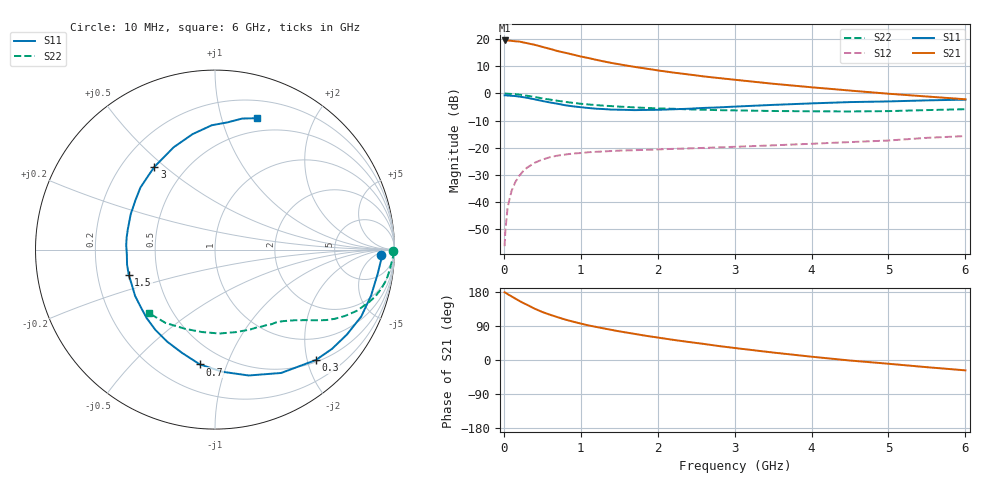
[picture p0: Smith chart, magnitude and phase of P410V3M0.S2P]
! SIEMENS Small Signal Semiconductors
! BFP182
! Si NPN RF Bipolar Junction Transistor in SOT143
! VCE = 10 V  IC = 3 mA
! Common Emitter S-Parameters:  March  1996
# GHz  S  MA  R  50
!  f  S11  S21  S12  S22
! GHz  MAG  ANG  MAG  ANG  MAG  ANG  MAG  ANG
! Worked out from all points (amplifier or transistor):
!   36 points, 10 MHz to 6 GHz, reference 50 ohm
!   highest |S21| = 19.6 dB at 10 MHz (marker M1)
!   |S21| within 3 dB of that: start of sweep to 585.2 MHz
!   unconditionally stable (mu >= 1): 2.001 GHz to 5.996 GHz
!   at 250 MHz: K = 0.16, MSG = 23.8 dB, |S12| = -28.8 dB
!   at 1.4 GHz: K = 0.76, MSG = 16.3 dB, |S12| = -21.3 dB
!   at 6 GHz: K = 1.00, MSG = 6.8 dB, |S12| = -15.8 dB
!   S11 on the Smith chart (normalised r, x): 10 MHz: 22, -8; 300 MHz: 0.54, -2.16; 700 MHz: 0.37, -0.81; 1.5 GHz: 0.34, -0.13; 3 GHz: 0.34, +0.46; 6 GHz: 0.36, +1.31
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0.01  0.9231 -1.7  9.558 178.6  0.0015 87.6  0.9934 -0.6
0.02  0.9275 -3.4  9.556 177.9  0.0029 89.3  0.9958 -1.4
0.05  0.9166 -8.4  9.554 173.8  0.008 87.0  0.9893 -3.3
0.1  0.9065 -16.5  9.401 167.9  0.0157 78.4  0.979 -6.8
0.2  0.8744 -32.7  9.133 156.1  0.0299 71.3  0.9519 -13.2
0.25  0.8549 -40.3  8.816 150.6  0.0365 67.1  0.9314 -16.2
0.3  0.8333 -47.6  8.517 145.9  0.0423 63.2  0.9088 -18.6
0.4  0.7799 -61.8  7.949 135.5  0.0522 56.6  0.8614 -23.3
0.5  0.7261 -75.0  7.28 126.7  0.06 50.1  0.8123 -27.1
0.6  0.682 -86.5  6.681 119.5  0.0663 45.5  0.7695 -30.1
0.7  0.6453 -97.5  6.085 112.9  0.071 41.5  0.7327 -32.4
0.8  0.6044 -107.6  5.647 106.6  0.0742 38.1  0.6991 -34.3
0.9  0.5781 -117.4  5.234 101.2  0.0776 35.6  0.6695 -36.0
1.1  0.5389 -135.0  4.52 91.3  0.0819 31.3  0.626 -38.9
1.5  0.5007 -163.8  3.468 75.6  0.0878 26.2  0.5717 -43.7
1.8  0.4953 177.2  2.954 65.4  0.0903 24.5  0.5439 -47.4
2.2  0.5094 157.2  2.438 53.2  0.0945 22.8  0.5212 -52.9
3  0.5715 126.2  1.795 31.7  0.1032 21.4  0.4867 -66.1
3.5  0.6149 112.0  1.512 19.7  0.1098 20.5  0.4741 -75.9
4.5  0.693 91.5  1.132 -1.4  0.1262 19.1  0.465 -99.0
5.5  0.7456 78.3  0.879 -19.0  0.1512 16.9  0.4926 -123.9
6  0.7688 72.2  0.781 -27.3  0.1631 13.7  0.5112 -136.3
